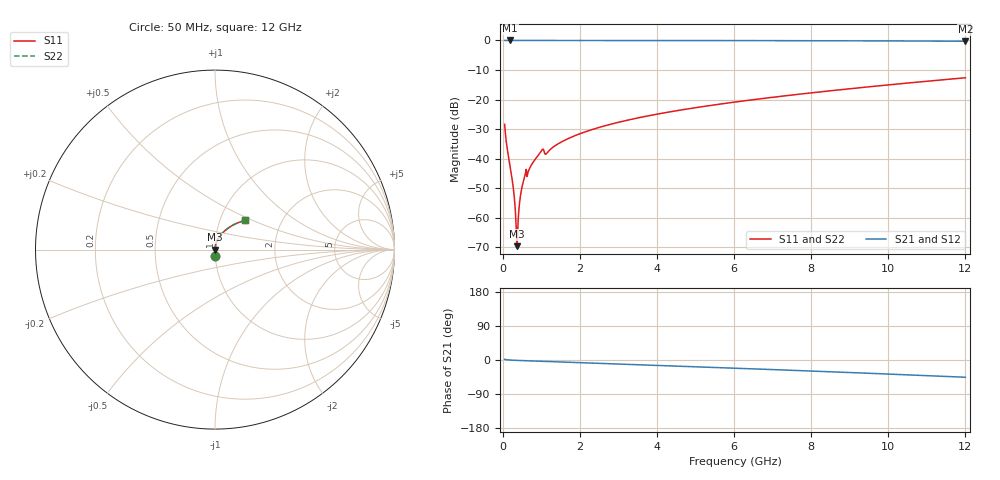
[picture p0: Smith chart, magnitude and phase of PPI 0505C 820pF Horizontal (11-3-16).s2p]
# MHz S MA R 50
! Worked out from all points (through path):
!   1601 points, 50 MHz to 12 GHz, reference 50 ohm
!   highest |S21| = 0.00 dB at 191.9 MHz (marker M1); lowest = -0.3 dB at 12 GHz (marker M2)
!   group delay of S21, straight-line fit = 10.5 ps
!   lowest |S11| = -69.6 dB at 371.2 MHz (marker M3), VSWR 1.00, Z = 50 + j0.000128 ohm
!   |S11| at or under -10 dB: start of sweep to end of sweep
!   |S22| runs from -69.6 to -12.6 dB; largest |S21 - S12| = 0
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50  0.03805 -87.7  0.9991 2.0  0.9991 2.0  0.03805 -87.7
87.34375  0.02097 -88.5  0.9996 1.0  0.9996 1.0  0.02097 -88.5
191.9062  0.007418 -88.0  0.9997 -0.1  0.9997 -0.1  0.007418 -88.0
266.5938  0.003542 -85.7  0.9997 -0.5  0.9997 -0.5  0.003542 -85.7
333.8125  0.001156 -74.9  0.9997 -0.9  0.9997 -0.9  0.001156 -74.9
371.1562  0.0003306 0.2  0.9996 -1.0  0.9996 -1.0  0.0003306 0.2
408.5  0.00108 70.3  0.9996 -1.2  0.9996 -1.2  0.00108 70.3
423.4375  0.001451 74.9  0.9996 -1.2  0.9996 -1.2  0.001451 74.9
453.3125  0.00218 79.2  0.9996 -1.4  0.9996 -1.4  0.00218 79.2
475.7188  0.002712 80.8  0.9996 -1.5  0.9996 -1.5  0.002712 80.8
557.875  0.004651 83.0  0.9995 -1.8  0.9995 -1.8  0.004651 83.0
849.1562  0.009862 84.1  0.9994 -2.9  0.9994 -2.9  0.009862 84.1
1013.469  0.01387 79.3  0.9981 -3.6  0.9981 -3.6  0.01387 79.3
1147.906  0.01245 79.1  0.9983 -3.9  0.9983 -3.9  0.01245 79.1
1484  0.01856 82.9  0.9991 -5.1  0.9991 -5.1  0.01856 82.9
2044.156  0.02701 81.5  0.9989 -7.2  0.9989 -7.2  0.02701 81.5
2910.531  0.03986 78.7  0.9983 -10.3  0.9983 -10.3  0.03986 78.7
4038.312  0.05717 74.9  0.9973 -14.3  0.9973 -14.3  0.05717 74.9
6025  0.09074 67.8  0.9945 -21.6  0.9945 -21.6  0.09074 67.8
8019.156  0.1302 60.3  0.9899 -29.2  0.9899 -29.2  0.1302 60.3
10013.31  0.1773 52.4  0.9822 -37.1  0.9822 -37.1  0.1773 52.4
12000  0.2337 44.1  0.97 -45.6  0.97 -45.6  0.2337 44.1
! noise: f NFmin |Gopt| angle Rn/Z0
50  0.0003041  0.8298  0.1755  0.0003763
1372  0.003079  0.5974  3.636  0.001405
2701  0.004546  0.4974  6.868  0.001555
4031  0.006066  0.4552  9.95  0.001853
5360  0.007513  0.428  12.87  0.002137
6682  0.008926  0.4101  15.62  0.002419
8012  0.01035  0.3988  18.25  0.002717
9341  0.01182  0.393  20.76  0.003041
1.067e+04  0.01335  0.3918  23.17  0.003403
1.2e+04  0.01498  0.3949  25.52  0.003818
